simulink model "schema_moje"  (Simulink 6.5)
settings: Solver=ode45  StartTime=0.0  StopTime=200.0  RelTol=1e-3
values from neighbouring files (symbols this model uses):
  A = [0 1 0 0;-P/M1 -D/M1 P/M1 0;0 0 0 1;P/M2 0 -P/M2 0]    [DED042_LQG.m]    (also in phinf2.m; podklad.m = [dh1_h10 dh1_h20 0; testx.m = [ -0.195 0.195; 0.195 -0.205]; kockaLQG.m = [0 1 0 0 0)
  B = [0;0;0;1/M2]    [DED042_LQG.m]    (also in phinf2.m; podklad.m = [dh1_q0; testx.m = [0.0047; 0]; kockaLQG.m = [0)
  C = [0 0 1 0]    [DED042_LQG.m]    (also in phinf2.m; podklad.m = [0 0 1]; testx.m = [0 1]; kockaLQG.m = [1 0 0 0 0])
  D = 0    [DED042_LQG.m]    (also in phinf2.m = [0]; podklad.m; testx.m = [0]; kockaLQG.m = [0])
  K = tf(num,den)    [phinf2.m]
  Ng = lqr_kompenzace(A,B,C,D,K)    [DED042_LQG.m]    (also in lqr_kompenzace.m = Nu + K*Nx; phinf2.m = -num(length(num))/den(length(den)); testx.m; kockaLQG.m)
undefined symbols (not defined in the file or in its folder): L

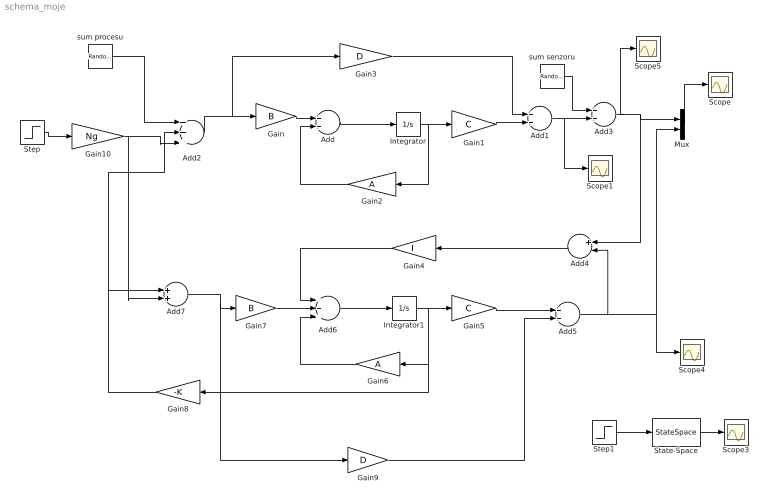
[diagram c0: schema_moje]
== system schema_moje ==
  Add{,1,3,5,7} (5 alike) : Sum  OutScaling=2^-10
  Add2 : Sum  Inputs=+++  OutScaling=2^-10
  Add4 : Sum  Orientation=left  Inputs=+-  OutScaling=2^-10
  Add6 : Sum  Inputs=+++  OutScaling=2^-10
  Gain : Gain  Gain=B  Multiplication=Matrix(K*u)
  Gain1 : Gain  Gain=C  Multiplication=Matrix(K*u)
  Gain10 : Gain  Gain=Ng
  Gain2 : Gain  Orientation=left  Gain=A  Multiplication=Matrix(K*u)
  Gain3 : Gain  Gain=D  Multiplication=Matrix(K*u)
  Gain4 : Gain  Orientation=left  Gain=L  Multiplication=Matrix(K*u)
  Gain5 : Gain  Gain=C  Multiplication=Matrix(K*u)
  Gain6 : Gain  Orientation=left  Gain=A  Multiplication=Matrix(K*u)
  Gain7 : Gain  Gain=B  Multiplication=Matrix(K*u)
  Gain8 : Gain  Orientation=left  Gain=-K  Multiplication=Matrix(K*u)
  Gain9 : Gain  Gain=D  Multiplication=Matrix(K*u)
  Integrator : Integrator
  Integrator1 : Integrator
  Mux : Mux  Inputs=2
  Scope{,1,3..5} (5 alike) : Scope
  State-Space : StateSpace  A=A  B=B  C=C  D=D
  Step : Step  Time=0  SampleTime=0
  Step1 : Step  SampleTime=0
  sum procesu : RandomNumber  Variance=0  SampleTime=0
  sum senzoru : RandomNumber  Variance=0  SampleTime=0
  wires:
  Integrator/1 -> Gain1/1, Gain2/1
  Gain/1 -> Add/1
  Add/1 -> Integrator/1
  Gain2/1 -> Add/2
  Add2/1 -> Gain/1, Gain3/1
  sum procesu/1 -> Add2/1
  Gain1/1 -> Add1/2
  Gain3/1 -> Add1/1
  Add1/1 -> Add3/2, Scope1/1
  sum senzoru/1 -> Add3/1
  Add3/1 -> Add4/1, Mux/1, Scope5/1
  Add5/1 -> Add4/2, Mux/2, Scope4/1
  Add4/1 -> Gain4/1
  Gain4/1 -> Add6/1
  Add6/1 -> Integrator1/1
  Integrator1/1 -> Gain5/1, Gain6/1, Gain8/1
  Gain5/1 -> Add5/1
  Gain6/1 -> Add6/3
  Gain7/1 -> Add6/2
  Gain8/1 -> Add2/2, Add7/1
  Step1/1 -> State-Space/1
  State-Space/1 -> Scope3/1
  Mux/1 -> Scope/1
  Gain9/1 -> Add5/2
  Add7/1 -> Gain7/1, Gain9/1
  Step/1 -> Gain10/1
  Gain10/1 -> Add2/3, Add7/2
